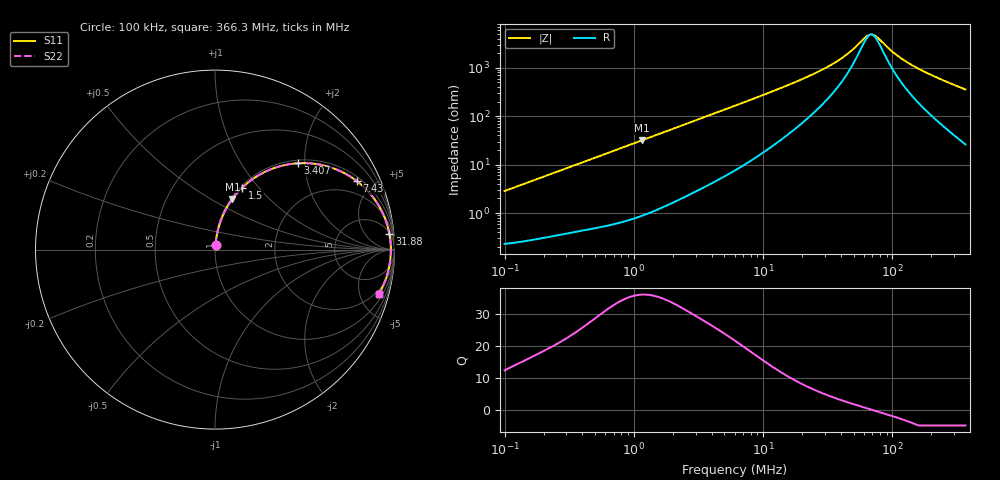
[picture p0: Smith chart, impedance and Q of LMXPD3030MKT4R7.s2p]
! LMXPD3030MKT4R7  S-PARAMETER MODEL  ( General Type )
! Model Generated by TAIYO YUDEN Corporation (https://www.yuden.co.jp/en/)
! Version 1.0
! TAIYO YUDEN Control No. 191023NI43SB-FBB
! Copyright(c) 2019 TAIYO YUDEN CO.,LTD. All Rights Reserved.
! Product Description (link to TY-COMPAS)
! https://ds.yuden.co.jp/TYCOMPAS/or/detail?pn=LMXPD3030MKT4R7M&u=M
! Products Name : Inductors
! Characteristics :
!  Inductance : 4.7 uH , SRF(min) : 48 MHz , DC Resistance(max) : 0.228 Ohm
!  Rated Current : Saturation :1250 mA , Temp Rise : 850 mA (40 degC)
!  Case Size : 3.0 x 3.0 / 0.118 x 0.118 [mm/inch] , Thickness : 1.2 / 0.047 [mm/inch]
!  (Conditions: Temperature = 25 degC , DC Bias Current/Voltage = 0A / 0V)
! External Node Assignments :
!  1  o---GGG---o  2
! GND o---------o GND
! Frequency Range : 0.1MHz  -  366.261039MHz  [ 402 STEP ]
# MHz S RI R 50
! Freq[MHz].  S11 Real  S11 Imag  S21 Real  S21 Imag  S12 Real  S12 Imag  S22 Real  S22 Imag
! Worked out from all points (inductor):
!   401 points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, 100 kHz to 366.3 MHz, reference 50 ohm
!   read as one part in series: L = 4.5 uH near 104.2 kHz
!   highest Q = 36.2 at 1.149 MHz (marker M1), where L = 4.37 uH
!   self-resonance near 68.59 MHz
!   S11 on the Smith chart (normalised r, x): 100 kHz: 1.00, +0.06; 1.5 MHz: 1.02, +0.82; 3.407 MHz: 1.07, +1.85; 7.43 MHz: 1.21, +4.04; 31.88 MHz: 6, +21; 366.3 MHz: 1.52, -7.11
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0.1  0.00309 0.0282  0.9969 -0.0282  0.9969 -0.0282  0.00309 0.0282
0.395307  0.016 0.1076  0.984 -0.1076  0.984 -0.1076  0.016 0.1076
1.148756  0.097 0.2825  0.903 -0.2825  0.903 -0.2825  0.097 0.2825
1.499861  0.1516 0.3448  0.8484 -0.3448  0.8484 -0.3448  0.1516 0.3448
1.562679  0.1619 0.3545  0.8381 -0.3545  0.8381 -0.3545  0.1619 0.3545
2.260687  0.2821 0.4349  0.7179 -0.4349  0.7179 -0.4349  0.2821 0.4349
3.407454  0.4637 0.4812  0.5363 -0.4812  0.5363 -0.4812  0.4637 0.4812
6.177387  0.7289 0.4218  0.2711 -0.4218  0.2711 -0.4218  0.7289 0.4218
7.430023  0.7917 0.3808  0.2083 -0.3808  0.2083 -0.3808  0.7917 0.3808
12.40872  0.9053 0.2566  0.0947 -0.2566  0.0947 -0.2566  0.9053 0.2566
23.92381  0.9622 0.1288  0.0378 -0.1288  0.0378 -0.1288  0.9622 0.1288
31.88328  0.9719 0.0871  0.0281 -0.0871  0.0281 -0.0871  0.9719 0.0871
43.37157  0.9773 0.0493  0.0227 -0.0493  0.0227 -0.0493  0.9773 0.0493
61.47043  0.9798 0.0114  0.0202 -0.0114  0.0202 -0.0114  0.9798 0.0114
66.72739  0.9799 0.00286  0.0201 -0.00286  0.0201 -0.00286  0.9799 0.00286
70.9631  0.9799 -0.00356  0.0201 0.00356  0.0201 0.00356  0.9799 -0.00356
75.46768  0.9798 -0.00999  0.0202 0.00999  0.0202 0.00999  0.9798 -0.00999
94.57258  0.9788 -0.034  0.0212 0.034  0.0212 0.034  0.9788 -0.034
118.514  0.9763 -0.0597  0.0237 0.0597  0.0237 0.0597  0.9763 -0.0597
157.9437  0.9704 -0.0965  0.0296 0.0965  0.0296 0.0965  0.9704 -0.0965
238.0629  0.9526 -0.1613  0.0474 0.1613  0.0474 0.1613  0.9526 -0.1613
366.261  0.9114 -0.2498  0.0886 0.2498  0.0886 0.2498  0.9114 -0.2498
